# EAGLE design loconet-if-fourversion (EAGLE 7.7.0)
Assembly variants: var1
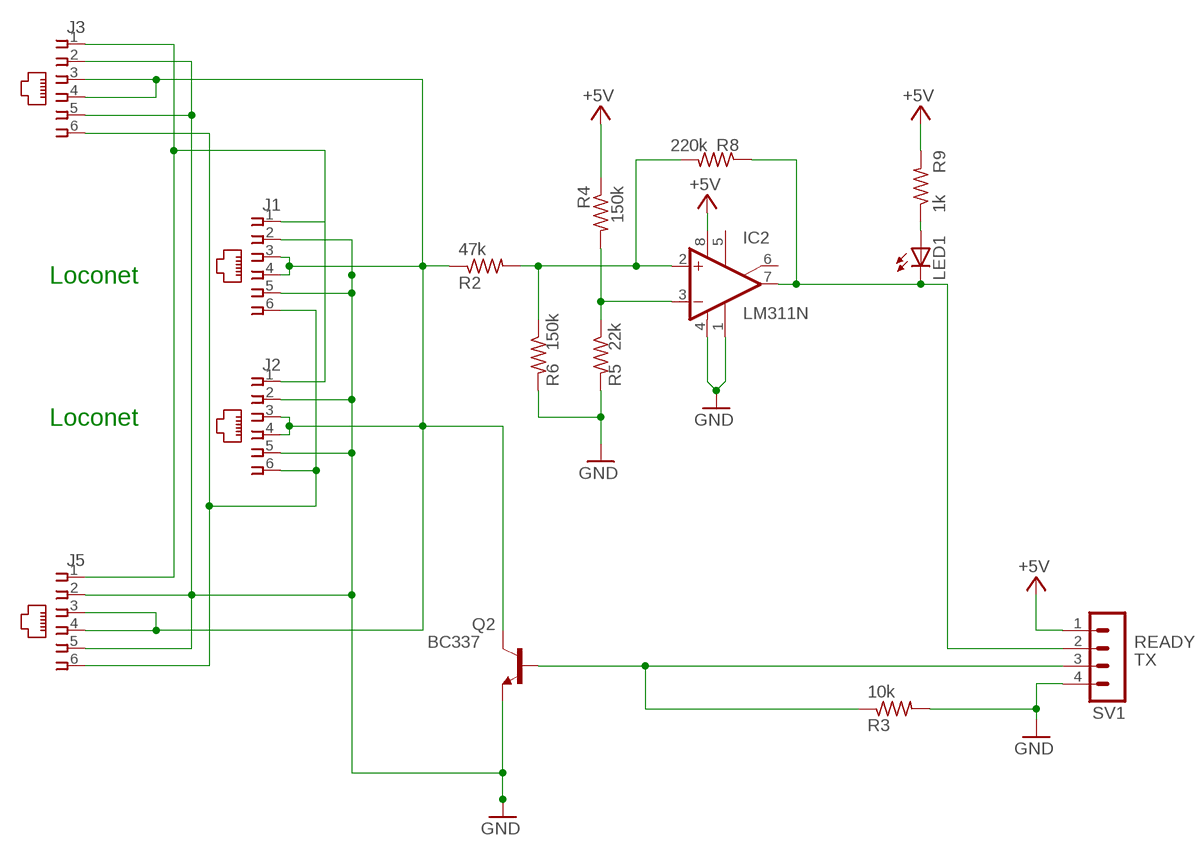
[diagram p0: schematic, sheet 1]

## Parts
IC2  LM311N  [DIL08]
J1  520425-3  [520425-3]
J2  520425-3  [520425-3]
J3  520425-3  [520425-3]
J5  520425-3  [520425-3]
LED1  LED3MM  [LED3MM]
Q2  BC337  2N3904  [TO92]
R2  47k  R-US_0204/7  [0204/7]
R3  10k  R-US_0204/7  [0204/7]
R4  150k  R-US_0204/7  [0204/7]
R5  22k  R-US_0204/7  [0204/7]
R6  150k  R-US_0204/7  [0204/7]
R8  220k  R-US_0204/7  [0204/7]
R9  1k  R-US_0204/7  [0204/7]
SV1  MA04-1  [MA04-1]

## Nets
+5V [power]: IC2.8(V+) R4.1 R9.2 SV1.1
GND: IC2.1(GND) IC2.4(V-) J1.2 J1.5 J2.2 J2.5 J3.2 J3.5 J5.2 J5.5 Q2.3(E) R3.2 R5.2 R6.2 SV1.4
N$1: LED1.A R9.1
N$3: J1.6 J2.6 J3.6 J5.6
N$6: J1.1 J2.1 J3.1 J5.1
N$14: IC2.2(+IN) R2.2 R6.1 R8.2
N$16: J1.3 J1.4 J2.3 J2.4 J3.3 J3.4 J5.3 J5.4 Q2.1(C) R2.1
N$17: IC2.3(-IN) R4.2 R5.1
READY: IC2.7(OUT) LED1.K(C) R8.1 SV1.2
TX: Q2.2(B) R3.1 SV1.3
Unconnected: IC2.5(ON) IC2.6(ON/STR)

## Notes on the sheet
- Loconet
- Loconet

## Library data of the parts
IC2 = linear:LM311: COMPARATOR
J1-J3 J5 = con-amp:520425-3: AMP connector
LED1 = led:LED: LED
Q2 = transistor-npn:2N3904: NPN Transistor
R2-R6 R8 R9 = rcl:R-US_: RESISTOR, American symbol
SV1 = con-lstb:MA04-1: PIN HEADER; OC_FARNELL: unknown; OC_NEWARK: unknown

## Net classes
0 default: width 0.457 mm
1 power: width 1.016 mm

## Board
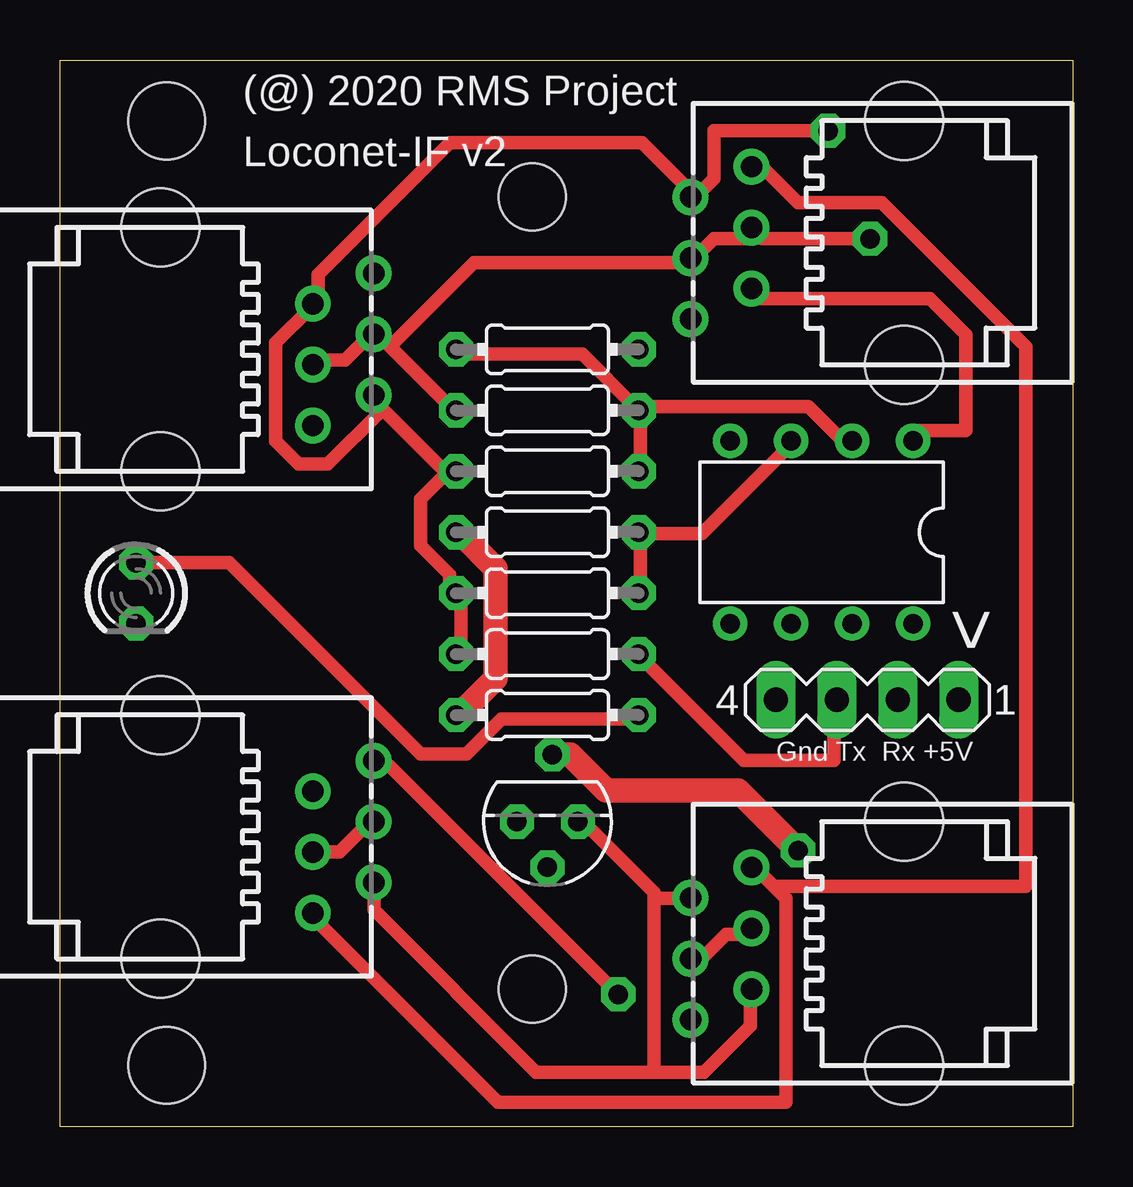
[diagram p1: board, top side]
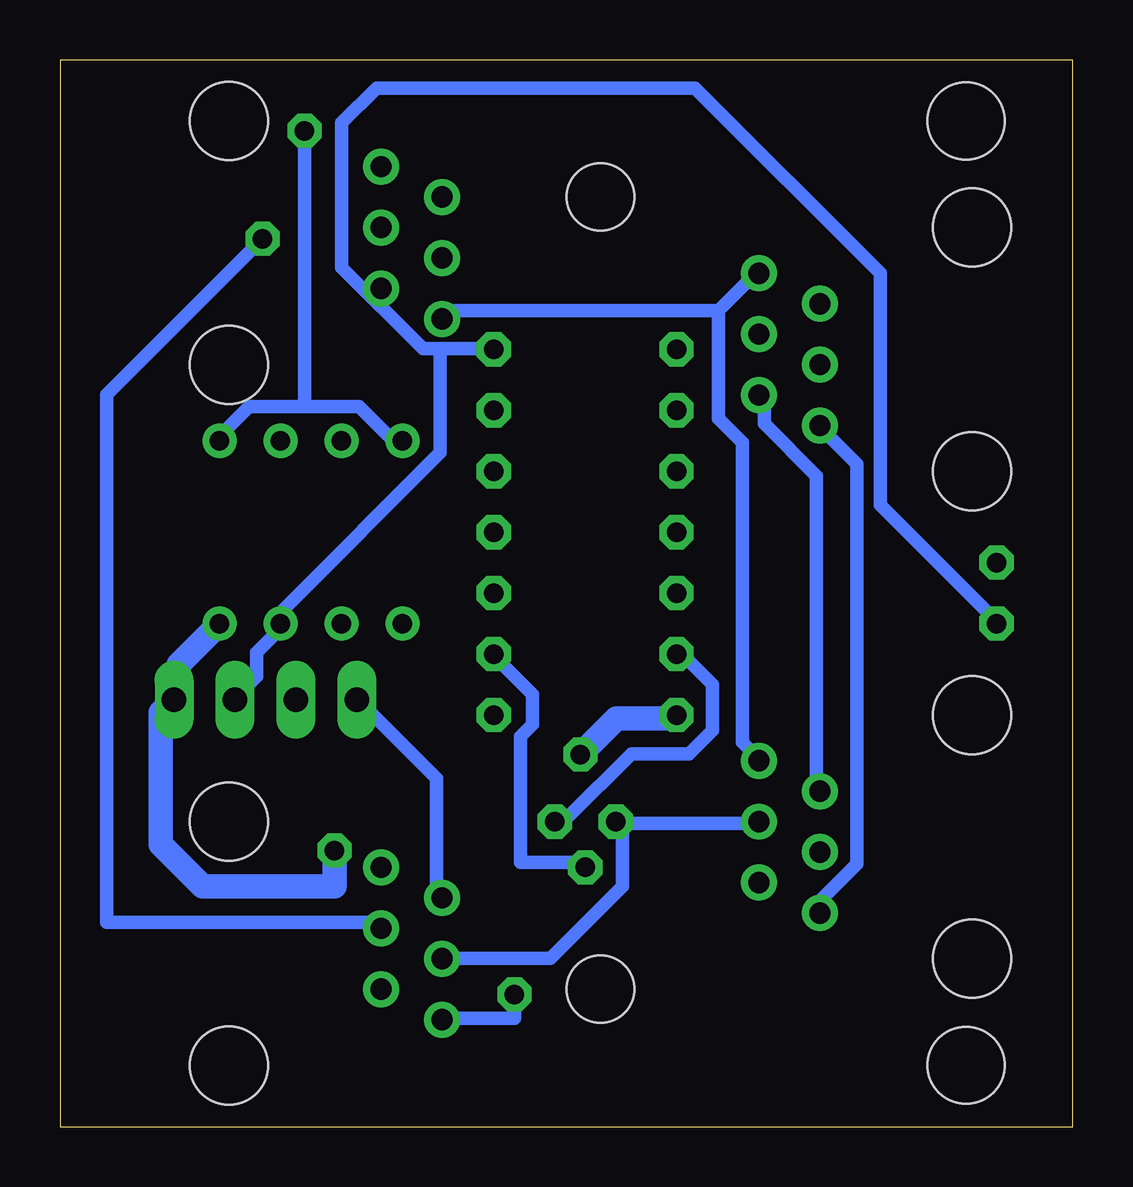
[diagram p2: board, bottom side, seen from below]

Size 42.22 x 44.46 mm. Coordinates in mm from the lower left corner, seen from the top.
Outline: 0,44.46 42.22,44.46 42.22,0 0,0 0,44.46
Copper layers (1*16): Top 0.02mm / dielectric 1.5mm / Bottom 0.02mm
Design rules "default *": minimum track width 22mil, minimum drill 32mil, track to track 16mil, track to pad 16mil, pad to pad 16mil, via to via 16mil, smd to smd 16mil, copper to edge 20mil, drill to drill 12mil, minimum pad ring 12mil, minimum via ring 12mil, stop-mask expansion 4mil, vias tented up to drill 0mil, thermal gap 10mil
Holes 2.8 mm at 19.68,5.72 19.68,38.74
Holes 3.2 mm at 4.45,41.92 4.45,2.55

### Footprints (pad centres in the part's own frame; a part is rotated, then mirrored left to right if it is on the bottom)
DIL08 = drill 0.813 pad 1.27: 1 -3.81,-3.81; 2 -1.27,-3.81; 3 1.27,-3.81; 4 3.81,-3.81; 5 3.81,3.81; 6 1.27,3.81; 7 -1.27,3.81; 8 -3.81,3.81
520425-3 = drill 0.889: 1 -3.175,8.001; 2 -1.905,5.461; 3 -0.635,8.001; 4 0.635,5.461; 5 1.905,8.001; 6 3.175,5.461 | hole 3.251: -5.08,-0.889; 5.08,-0.889
LED3MM = drill 0.813 octagon: A -1.27,0; K 1.27,0
TO92 = drill 0.813 octagon: 1 1.27,0; 2 0,1.905; 3 -1.27,0
0204/7 = drill 0.813 octagon: 1 -3.81,0; 2 3.81,0
MA04-1 = drill 1.016 long: 1 -3.81,0; 2 -1.27,0; 3 1.27,0; 4 3.81,0

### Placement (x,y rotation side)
IC2  31.75,24.78 180 top
J1  5.08,12.07 270 top
J2  5.08,32.39 270 top
J3  34.29,7.63 90 top
J5  34.29,36.84 90 top
LED1  3.17,22.24 270 top
Q2  20.32,12.71 180 top
R2  20.32,29.86 0 top
R3  20.32,19.7 180 top
R4  20.32,24.78 0 top
R5  20.32,22.24 180 top
R6  20.32,27.32 180 top
R8  20.32,32.39 180 top
R9  20.32,17.16 180 top
SV1  33.66,17.79 180 top

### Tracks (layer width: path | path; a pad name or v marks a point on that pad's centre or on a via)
+5V  (via drill 0.81)
  Top 1.016: R9.2 16.71,17.23 18.16,18.68 18.16,23.26 16.71,24.71 R4.1 | v30.77,11.51 28.27,14.01 22.77,14.01 21.27,15.51 v20.52,15.51
  Bottom 1.016: IC2.8 35.77,20.76 37.27,19.26 37.27,18.01 SV1.1 37.77,17.51 38.02,17.26 38.02,11.76 36.27,10.01 30.77,10.01 v30.77,11.51 | v20.52,15.51 19.02,17.01 16.52,17.01 R9.2
GND  (via drill 0.81)
  Top 0.559: 24.77,2.27 26.85,2.27 28.78,4.2 28.78,4.92 J3.2 | 24.77,2.27 19.85,2.27 13.09,9.03 13.09,9.99 J1.5 | R3.2 16.71,19.89 16.71,22.06 R5.2 16.23,22.3 16.23,23.02 15.02,24.23 15.02,26.16 15.99,27.12 R6.2 16.47,27.37 15.99,27.37 13.09,30.26 J2.5 13.34,29.78 11.16,27.61 9.96,27.61 8.99,28.57 8.99,32.67 10.44,34.12 J2.2 10.77,34.51 10.77,35.51 16.27,41.01 24.27,41.01 26.27,39.01 J5.5 26.52,38.76 27.27,39.51 27.27,41.51 v32.02,41.51 | J5.2 29.27,34.51 36.27,34.51 37.77,33.01 37.77,29.01 35.77,29.01 IC2.1 | 24.77,9.51 24.77,2.27 | 24.77,9.51 26.27,9.51 J3.5 | 24.77,9.51 24.77,9.76 22.02,12.51 21.77,12.51 Q2.3
  Bottom 0.559: 32.02,30.02 34.33,30.02 35.53,28.81 IC2.1 | 32.02,30.02 29.74,30.02 28.54,28.81 28.05,28.81 IC2.4 | J1.2 10.68,14.09 10.68,27.12 12.85,29.3 12.85,30.26 J2.5 | Q2.3 21.54,12.89 21.06,12.89 18.4,15.54 15.99,15.54 15.02,16.51 15.02,18.44 16.23,19.64 R3.2 | SV1.4 29.77,17.76 26.52,14.51 26.52,9.76 J3.5 | 32.02,30.02 v32.02,41.51
N$1
  Top 0.559: LED1.A 7.06,23.51 15.02,15.54 16.95,15.54 18.4,16.99 23.95,16.99 R9.1
N$3
  Top 0.559: 29.77,10.01 30.27,9.51 30.27,1.01 18.27,1.01 10.77,8.51 J1.6 | 29.77,10.01 29.27,10.51 J3.6 | 29.77,10.01 40.27,10.01 40.27,32.51 34.27,38.51 30.77,38.51 29.27,40.01 J5.6
  Bottom 0.559: J1.6 10.44,9.03 10.44,9.51 8.99,10.96 8.99,27.61 10.44,29.06 J2.6
N$6  (via drill 0.81)
  Top 0.559: v23.27,5.51 13.77,15.01 13.27,15.01 J1.1
  Bottom 0.559: 14.77,34.01 14.77,29.51 13.77,28.51 13.77,16.01 13.27,15.51 J1.1 | 14.77,34.01 13.27,35.51 J2.1 | v23.27,5.51 23.27,4.51 26.27,4.51 J3.1 | 14.77,34.01 26.27,34.01 J5.1
N$14
  Top 0.559: R6.1 24.19,27.37 24.19,29.78 R2.2 | IC2.2 32.88,28.81 32.4,28.81 31.19,30.02 24.19,30.02 R2.2 | R8.2 16.71,32.19 21.78,32.19 23.95,30.02 R2.2
N$16  (via drill 0.81)
  Top 0.559: J1.4 11.65,11.44 12.85,12.65 J1.3 | J2.4 10.68,31.95 11.89,31.95 12.85,32.92 J2.3 13.27,33.01 13.77,32.51 | J3.3 26.77,7.01 27.77,8.01 28.77,8.01 J3.4 | 13.77,32.51 16.27,30.01 R2.1 | 13.77,32.51 17.27,36.01 26.27,36.01 J5.3 26.77,36.51 27.27,37.01 28.77,37.01 J5.4 29.27,37.01 v33.77,37.01
  Bottom 0.559: J1.3 13.09,12.65 18.89,12.65 Q2.1 18.77,12.51 18.77,10.01 21.77,7.01 26.27,7.01 J3.3 | v33.77,37.01 40.27,30.51 40.27,8.51 29.27,8.51 J3.4
N$17
  Top 0.559: R5.1 24.19,22.3 24.19,24.71 R4.2 24.43,24.71 26.76,24.71 30.62,28.57 30.47,28.57 IC2.3
READY
  Bottom 0.559: 26.36,32.43 24.19,32.43 R8.1 | 26.36,32.43 27.09,32.43 30.47,35.81 30.47,41.84 29.02,43.29 15.75,43.29 8.03,35.57 8.03,25.92 3.2,21.09 LED1.K | 26.36,32.43 26.36,28.09 32.88,21.58 32.88,21.09 IC2.7 33.02,20.76 34.02,19.76 34.02,18.76 34.77,18.01 SV1.2
TX
  Top 0.559: SV1.3 32.27,17.76 32.27,15.26 28.52,15.26 24.27,19.51 R3.1
  Bottom 0.559: Q2.2 20.52,11.01 23.02,11.01 23.02,16.26 22.52,16.76 22.52,18.01 24.02,19.51 R3.1

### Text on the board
tNames: (@) 2020 RMS Project | Loconet-IF v2 | < | Gnd Tx Rx +5V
